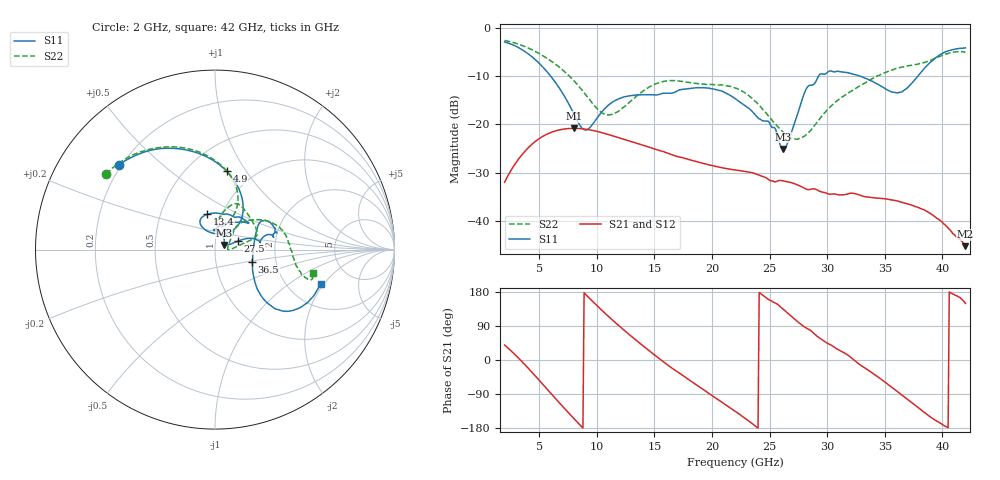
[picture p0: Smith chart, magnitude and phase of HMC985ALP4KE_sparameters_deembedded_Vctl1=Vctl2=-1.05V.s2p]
!s2p File: Measurements: S11, S21, S12, S22
# GHz S dB R 50.0
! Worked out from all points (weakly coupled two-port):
!   401 points, 2 GHz to 42 GHz, reference 50 ohm
!   highest |S21| = -20.80 dB at 8 GHz (marker M1); lowest = -45.2 dB at 42 GHz (marker M2)
!   lowest |S11| = -25.0 dB at 26.2 GHz (marker M3), VSWR 1.12, Z = 55.2 + j2.8 ohm
!   |S11| at or under -10 dB: 5.999 GHz to 29.25 GHz (23.25 GHz wide, 132 % of centre); 32.83 GHz to 37.87 GHz (5.04 GHz wide, 14.3 % of centre)
!   |S22| runs from -23.1 to -2.6 dB; largest |S21 - S12| = 0.00015
!   S11 on the Smith chart (normalised r, x): 2 GHz: 0.19, +0.37; 4.9 GHz: 0.76, +0.82; 13.4 GHz: 0.85, +0.35; 27.5 GHz: 1.29, +0.12; 36.5 GHz: 1.50, -0.21; 42 GHz: 3.02, -1.86
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2  -2.92 138.7  -31.95 39.5  -31.96 39.5  -2.62 145.2
3.4  -4.37 111.3  -26.57 -0.8  -26.58 -0.8  -3.55 122.5
4.9  -7.11 81.5  -23.09 -49.9  -23.10 -49.9  -5.19 99.1
6.3  -10.94 56.5  -21.41 -97.7  -21.42 -97.7  -7.33 79.6
8  -17.75 49.6  -20.80 -154.1  -20.81 -154.2  -10.91 63.7
8.7  -20.71 68.9  -20.88 -176.4  -20.89 -176.4  -12.84 61.6
10.9  -16.23 120.0  -22.00 118.2  -22.00 118.2  -18.00 78.9
13.4  -13.90 102.1  -23.83 52.6  -23.84 52.5  -14.23 80.5
15.4  -13.78 75.2  -25.34 4.5  -25.34 4.5  -11.34 68.4
18.9  -12.41 39.4  -27.83 -70.8  -27.84 -70.8  -11.58 41.4
22  -14.62 55.0  -29.39 -135.0  -29.40 -135.0  -12.42 17.5
24.9  -19.36 90.1  -31.34 159.9  -31.35 159.9  -18.21 8.3
26.2  -25.05 26.9  -31.67 133.4  -31.68 133.4  -21.64 0.1
27.5  -17.33 20.2  -32.59 99.6  -32.59 99.6  -22.97 5.9
28.2  -12.58 14.1  -33.39 84.2  -33.37 84.1  -22.11 18.3
28.7  -11.84 9.2  -33.33 74.5  -33.33 74.5  -20.82 27.1
31  -9.02 20.1  -34.56 26.7  -34.53 26.8  -14.83 47.3
33.3  -10.41 31.5  -34.94 -21.5  -34.95 -21.6  -11.38 37.9
35.4  -13.05 10.5  -35.52 -67.2  -35.50 -67.2  -8.93 23.8
36.5  -13.25 -18.0  -36.12 -92.8  -36.12 -92.9  -8.11 15.4
39.6  -5.92 -42.5  -39.51 -162.8  -39.48 -162.7  -6.09 -15.3
42  -4.15 -17.9  -45.16 149.4  -45.12 149.4  -5.02 -13.4
